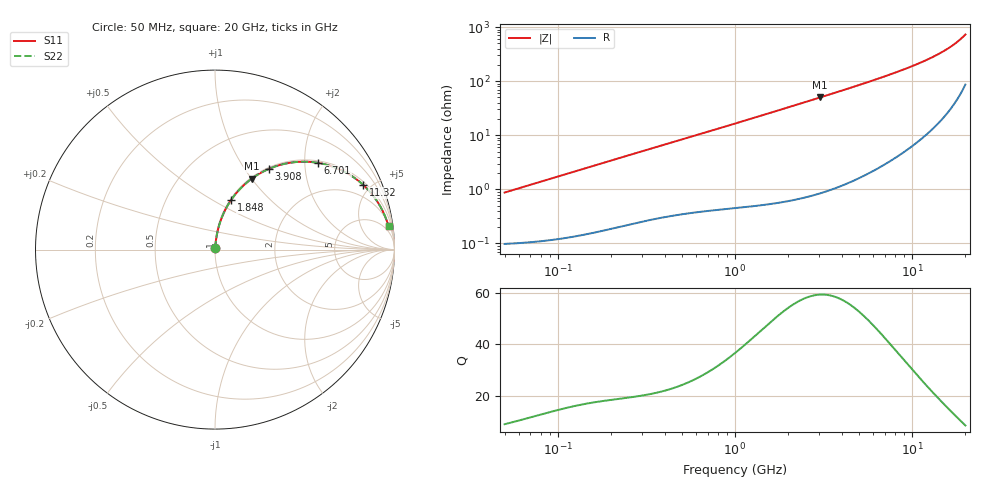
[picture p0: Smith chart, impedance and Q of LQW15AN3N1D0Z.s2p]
!Murata Part Number: LQW15AN3N1D0Z
!These Parameters are Measured in Series Mode Connection
!  o--[Z]--o
!Port1  Port2
!  o-------o
!Freq. Start=50[MHz] Stop=20[GHz], 401[Steps]
# Hz S RI R 50
!Freq.(Hz) S11(Real) S11(Imag) S21(Real) S21(Imag) S12(Real) S12(Imag) S22(Real) S22(Imag)
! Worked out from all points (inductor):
!   401 points, 50 MHz to 20 GHz, reference 50 ohm
!   read as one part in series: L = 2.76 nH near 51.52 MHz
!   highest Q = 59.3 at 3.03 GHz (marker M1), where L = 2.63 nH
!   S11 on the Smith chart (normalised r, x): 50 MHz: 1.00, +0.02; 1.848 GHz: 1.01, +0.61; 3.908 GHz: 1.02, +1.30; 6.701 GHz: 1.05, +2.33; 11.32 GHz: 1.17, +4.49; 20 GHz: 3, +14
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5e7  0.00105 0.00866  0.9989 -0.00866  0.9989 -0.00866  0.00105 0.00866
1.364002e8  0.00197 0.0234  0.998 -0.0234  0.998 -0.0234  0.00197 0.0234
3.721004e8  0.00677 0.0618  0.9932 -0.0618  0.9932 -0.0618  0.00677 0.0618
6.285508e8  0.0144 0.1021  0.9856 -0.1021  0.9856 -0.1021  0.0144 0.1021
1e9  0.0304 0.1586  0.9696 -0.1586  0.9696 -0.1586  0.0304 0.1586
1.390315e9  0.0538 0.2147  0.9462 -0.2147  0.9462 -0.2147  0.0538 0.2147
1.848039e9  0.0886 0.2748  0.9114 -0.2748  0.9114 -0.2748  0.0886 0.2748
2.245319e9  0.1243 0.3212  0.8757 -0.3212  0.8757 -0.3212  0.1243 0.3212
2.728004e9  0.1725 0.3694  0.8275 -0.3694  0.8275 -0.3694  0.1725 0.3694
3.029571e9  0.2045 0.395  0.7955 -0.395  0.7955 -0.395  0.2045 0.395
3.908127e9  0.301 0.4501  0.699 -0.4501  0.699 -0.4501  0.301 0.4501
5.194772e9  0.4377 0.4865  0.5623 -0.4865  0.5623 -0.4865  0.4377 0.4865
5.944466e9  0.5094 0.4896  0.4906 -0.4896  0.4906 -0.4896  0.5094 0.4896
6.701223e9  0.5743 0.4832  0.4257 -0.4832  0.4257 -0.4832  0.5743 0.4832
7.442007e9  0.6303 0.4705  0.3697 -0.4705  0.3697 -0.4705  0.6303 0.4705
9.041845e9  0.7284 0.4302  0.2716 -0.4302  0.2716 -0.4302  0.7284 0.4302
1.131968e10  0.8251 0.3611  0.1749 -0.3611  0.1749 -0.3611  0.8251 0.3611
1.334722e10  0.8816 0.2997  0.1184 -0.2997  0.1184 -0.2997  0.8816 0.2997
1.550395e10  0.9219 0.2388  0.0781 -0.2388  0.0781 -0.2388  0.9219 0.2388
1.747767e10  0.9466 0.1879  0.0534 -0.1879  0.0534 -0.1879  0.9466 0.1879
1.940974e10  0.9629 0.1425  0.0371 -0.1425  0.0371 -0.1425  0.9629 0.1425
2e10  0.9667 0.1294  0.0333 -0.1294  0.0333 -0.1294  0.9667 0.1294
